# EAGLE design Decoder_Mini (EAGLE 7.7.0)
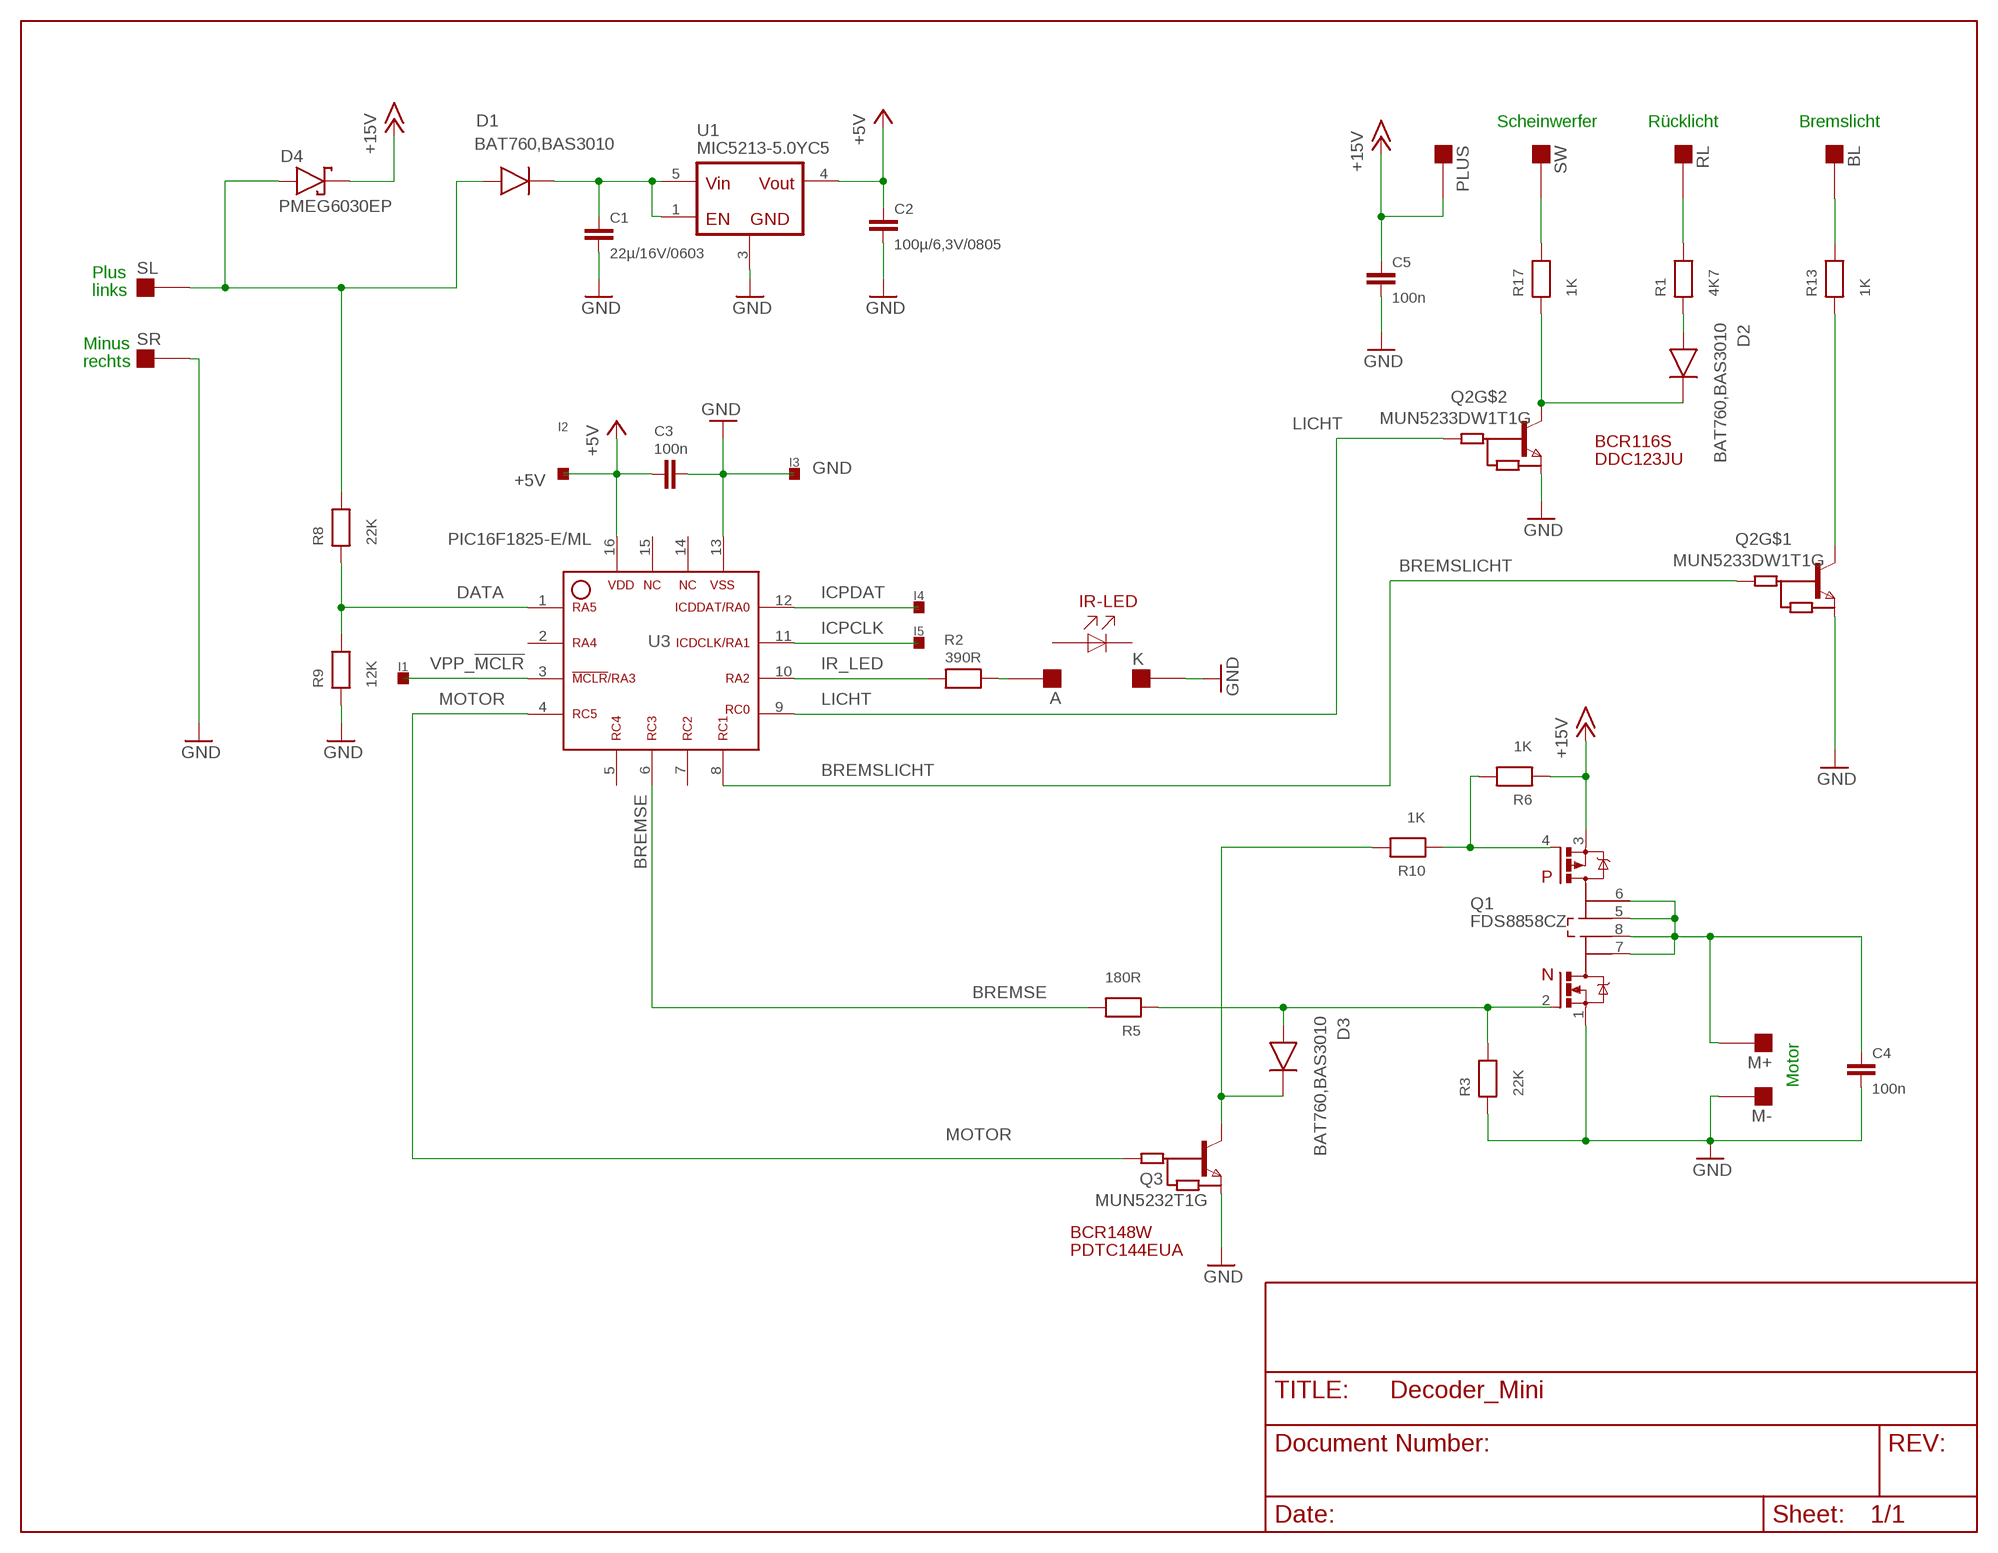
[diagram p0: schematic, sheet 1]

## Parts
A  A  LOETPAD1.5  [LOETPAD_RUND]
BL  LOETPAD_1.6X1.6_MM  [LOETPAD_1.6X1.6_MM]
C1  22µ/16V/0603  C-0603R  [0603-R]
C2  100µ/6,3V/0805  C-0805R  [0805-R]
C3  100n  C-0402R  [0402-R]
C4  100n  C-0402R  [0402-R]
C5  100n  C-0402R  [0402-R]
D1  BAT760,BAS3010  BAR65-03WBIG  [SOD323_BIG]
D2  BAT760,BAS3010  BAR65-03WBIG  [SOD323_BIG]
D3  BAT760,BAS3010  BAR65-03WBIG  [SOD323_BIG]
D4  PMEG6030EP  [SOD128]
I1  INCIR-PADOVAL  [TEST_PAD_OVAL]
I2  INCIR-PADOVAL  [TEST_PAD_OVAL]
I3  INCIR-PADOVAL  [TEST_PAD_OVAL]
I4  INCIR-PADOVAL  [TEST_PAD_OVAL]
I5  INCIR-PADOVAL  [TEST_PAD_OVAL]
K  K  LOETPAD1.5  [LOETPAD_RUND]
M+  LOETPAD_2X2MM  [LOETPAD_2X2_MM]
M-  LOETPAD_2X2MM  [LOETPAD_2X2_MM]
PLUS  LOETPAD_1.6X1.6_MM  [LOETPAD_1.6X1.6_MM]
Q1  FDS8858CZ  SI4501BDY  [SO8_COOLING]
Q2  MUN5233DW1T1G  DDC123JUSOT363-3  [SOT363-6]
Q3  MUN5232T1G  PDTC144EUFRANK  [SC70_FRANK]
R1  4K7  RES-0402W  [0402-W]
R2  390R  RES-0402R  [0402-R]
R3  22K  RES-0402R  [0402-R]
R5  180R  RES-0402W  [0402-W]
R6  1K  RES-0402W  [0402-W]
R8  22K  RES-0402R  [0402-R]
R9  12K  RES-0402R  [0402-R]
R10  1K  RES-0402W  [0402-W]
R13  1K  RES-0402W  [0402-W]
R17  1K  RES-0402W  [0402-W]
RL  LOETPAD_1.6X1.6_MM  [LOETPAD_1.6X1.6_MM]
SL  LOETPAD_2X2MM  [LOETPAD_2X2_MM]
SR  LOETPAD_2X2MM  [LOETPAD_2X2_MM]
SW  LOETPAD_1.6X1.6_MM  [LOETPAD_1.6X1.6_MM]
U1  MIC5213-5.0YC5  MIC5213  [SOT363-5]
U3  PIC16F1825-E/ML  PIC16F182X/ML  [QFN_4X4X0.9]

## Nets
+5V: C2.1 C3.1 I2.1 U1.4(VOUT) U3.16
+15V: C5.1 D4.K PLUS.P$1 Q1.3(S2) R6.1
AN: A.P$1 R2.1
BREMSE: R5.2 U3.6
BREMSLICHT: Q2.2(B) U3.8
D!: D2.K Q2.3(C) R17.1
DATA: R8.1 R9.2 U3.1
GND: C1.2 C2.2 C3.2 C4.2 C5.2 I3.1 K.P$1 M-.P$1 Q1.1(S1) Q2.1(E) Q2.4(E) Q3.2(E) R3.1 R9.1 SR.P$1 U1.3(GND) U3.13
ICPCLK: I5.1 U3.11
ICPDAT: I4.1 U3.12
IR_LED: R2.2 U3.10
LICHT: Q2.5(B) U3.9
M_PLUS: C4.1 M+.P$1 Q1.5(D2A) Q1.6(D2B) Q1.7(D1A) Q1.8(D1B)
MOTOR: Q3.1(B) U3.4
N$1: C1.1 D1.K U1.1(EN) U1.5(VIN)
N$4: BL.P$1 R13.2
N$6: D1.A D4.A R8.2 SL.P$1
N$7: R1.2 RL.P$1
N$8: D2.A R1.1
N$9: R17.2 SW.P$1
N$11: D3.A Q1.2(G1) R3.2 R5.1
N$13: Q2.6(C) R13.1
N$16: D3.K Q3.3(C) R10.2
N$17: Q1.4(G2) R6.2 R10.1
VPP_!MCLR!: I1.1 U3.3
Unconnected: U3.2 U3.5 U3.7 U3.14 U3.15

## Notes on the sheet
- Scheinwerfer | Rücklicht | Bremslicht
- Plus
- links
- Minus
- rechts
- BCR116S
- DDC123JU
- IR-LED
- Motor
- BCR148W
- PDTC144EUA

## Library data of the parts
A K = Hobby:LOETPAD: Lötpad
BL PLUS RL SW = Hobby:LOETPAD_1.6X1.6_MM: Lötpad 1,6 x 1,6 mm, Bohrung 0,7mm
C1-C5 = RCL:C: Kondensatoren CM 2003
D1-D3 = SMD:BAR65-03W*
D4 = Hobby:PMEG6030EP: 3 A low VF MEGA Schottky barrier rectifier
I1-I5 = SMD:INCIR-PAD*
M+ M- SL SR = Hobby:LOETPAD_2X2MM: Lötpad 2 x 2 mm mit Durchkontaktierung
Q1 = Hobby:SI4501BDY: Complementary N and P Channel MOSFET
Q2 = Hobby:DDC123JU*: NPN PRE-BIASED SMALL SIGNAL DUAL SURFACE MOUNT TRANSISTOR
Q3 = Hobby:PDTC144EU*: NPN Transistor mit Vorwiderständen
R1-R3 R5 R6 R8-R10 R13 R17 = RCL:RES: Widerstand
U1 = Hobby:MIC5213: Teeny™ SC-70 μCap Low-Dropout Regulator
U3 = Hobby:PIC16F182X*: Microchip 8 Bit µC

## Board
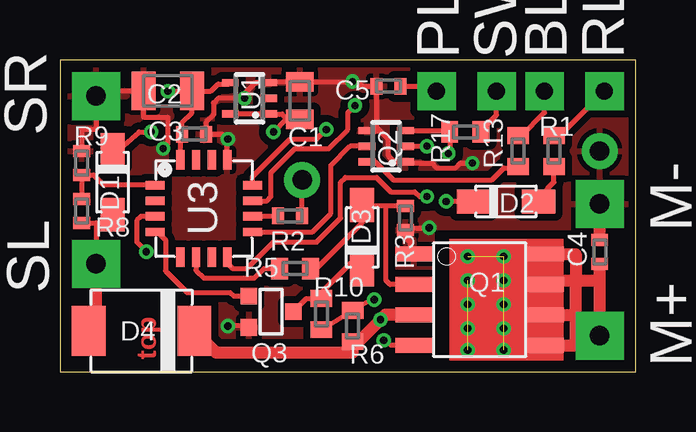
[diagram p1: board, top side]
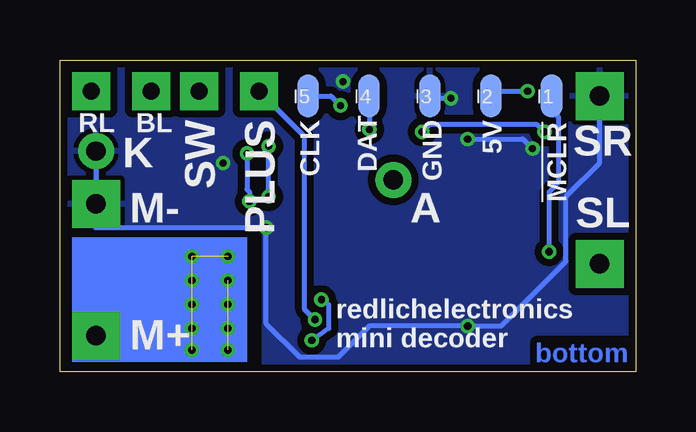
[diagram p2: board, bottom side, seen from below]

Size 24 x 13 mm. Coordinates in mm from the lower left corner, seen from the top.
Outline: 0,0 24,0 24,13 0,13 0,0
Copper layers (1*16): Top 0.035mm / dielectric 1.5mm / Bottom 0.035mm
Design rules "PCB-POOL Standard *": minimum track width 0.15mm, minimum drill 0.3mm, track to track 0.15mm, track to pad 0.15mm, pad to pad 0.15mm, via to via 0.15mm, smd to smd 0.15mm, copper to edge 0.3mm, drill to drill 0.2mm, minimum pad ring 0.2mm, minimum via ring 0.15mm, stop-mask expansion 0.075mm, vias tented up to drill 0.5mm, thermal gap 0.2mm

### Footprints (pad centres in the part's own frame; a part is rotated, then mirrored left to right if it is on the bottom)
LOETPAD_RUND = drill 0.8 pad 1.5: P$1 0,0
LOETPAD_1.6X1.6_MM = drill 0.7 pad 1.6 square: P$1 0,0
0603-R = smd 0.813 x 1.143: 1 -0.787,0; 2 0.787,0
0805-R = smd 0.991 x 1.6: 1 -1.016,0; 2 1.016,0
0402-R = smd 0.5 x 0.7: 1 -0.5,0; 2 0.5,0
SOD323_BIG = smd 1.4 x 1: A 1.35,0; K -1.35,0
SOD128 = smd 1.4 x 2.1: A -2.2,0; K 2.2,0
TEST_PAD_OVAL = smd 0.9 x 1.8: 1 0,0
LOETPAD_2X2_MM = drill 0.8 pad 2 square: P$1 0,0
SO8_COOLING = smd 0.61 x 1.524: 1 -1.905,-2.743; 2 -0.635,-2.743; 3 0.635,-2.743; 4 1.905,-2.743; 5 1.905,2.743; 6 0.635,2.743; 7 -0.635,2.743; 8 -1.905,2.743
SOT363-6 = smd 0.3 x 0.7: 1 -0.65,-0.8; 2 0,-0.8; 3 0.65,-0.8; 4 0.65,0.8; 5 0,0.8; 6 -0.65,0.8
SC70_FRANK = smd 0.7 x 0.7: 1 -0.65,-0.925; 2 0.65,-0.925; 3 0,0.925
0402-W = smd 0.7 x 0.9: 1 -0.65,0; 2 0.65,0
SOT363-5 = smd 0.3 x 0.7: 1 -0.65,-0.8; 2 0,-0.8; 3 0.65,-0.8; 4 0.65,0.8; 5 -0.65,0.8
QFN_4X4X0.9 = smd 0.35 x 0.8: 1 -0.975,-2.031; 2 -0.325,-2.031; 3 0.325,-2.031; 4 0.975,-2.031; 9 0.975,2.031; 10 0.325,2.031; 11 -0.325,2.031; 12 -0.975,2.031 | smd 0.8 x 0.35: 5 2.031,-0.975; 6 2.031,-0.325; 7 2.031,0.325; 8 2.031,0.975; 13 -2.031,0.975; 14 -2.031,0.325; 15 -2.031,-0.325; 16 -2.031,-0.975

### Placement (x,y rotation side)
A  10.1,8 0 top
BL  20.2,11.7 0 top
C1  10,11.3 90 top
C2  4.5,11.7 180 top
C3  5.6,9.9 0 top
C4  22.5,5 90 top
C5  13.7,11.9 180 top
D1  2.2,7.9 270 top
D2  18.6,7.1 0 top
D3  12.6,5.6 90 top
D4  3.4,1.7 0 top
I1  3.5,11.5 0 bottom
I2  6.04,11.5 0 bottom
I3  8.58,11.5 0 bottom
I4  11.12,11.5 0 bottom
I5  13.66,11.5 0 bottom
K  22.5,9.2 0 top
M+  22.5,1.5 270 top
M-  22.5,7 270 top
PLUS  15.7,11.7 0 top
Q1  17.5,3 270 top
Q2  13.6,9.4 90 top
Q3  8.8,2.5 270 top
R1  20.6,9.2 90 top
R2  9.6,6.5 180 top
R3  14.4,6.4 90 top
R5  9.8,4.3 180 top
R6  12.2,1.9 90 top
R8  0.9,6.7 270 top
R9  0.9,8.7 270 top
R10  10.9,2.4 90 top
R13  19.1,9.2 90 top
R17  16.9,10 0 top
RL  22.7,11.7 0 top
SL  1.5,4.5 0 top
SR  1.5,11.5 0 top
SW  18.2,11.7 0 top
U1  7.9,11.4 90 top
U3  6,6.8 270 top

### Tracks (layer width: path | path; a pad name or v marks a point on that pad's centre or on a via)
+5V  (via drill 0.3)
  Top 0.2: v4.5,11.7 C2.1 | C2.1 6.3,11.7 6.6,12 7.05,12 U1.4 | C2.1 5.5,11.68 5.5,10.8 5.1,10.4 C3.1 5.03,9.82 U3.16
  Bottom 0.2: I2.1 5.84,11.7 v4.5,11.7
+15V  (via drill 0.3)
  Top 0.2: C5.1 15.5,11.9 PLUS.P$1
  Top 0.5: D4.K 6.5,0.8 12.2,0.8 R6.1 12.45,1.25 v13.37,2.17 13.56,2.37 Q1.3
  Bottom 0.2: v13.37,2.17 13.8,2.6 13.8,9.8 PLUS.P$1
AN
  Top 0.2: R2.1 A.P$1
BREMSE
  Top 0.2: U3.6 5.67,4.22 6,3.9 8.1,3.9 8.5,4.3 R5.2
BREMSLICHT  (via drill 0.3)
  Top 0.2: U3.8 7.03,4.47 7.2,4.3 7.8,4.3 8.9,5.4 10.7,5.4 11.7,6.4 11.7,7.9 11.9,8.1 13.2,8.1 13.8,7.5 14.8,7.5 15,7.3 v15.3,7.3 | Q2.2 v15.3,9.4
  Bottom 0.2: v15.3,7.3 v15.3,9.4
D!  (via drill 0.3)
  Top 0.2: Q2.3 16.2,10.05 R17.1 16.25,9.25 v16.2,9.1 | D2.K v16.1,7.1
  Bottom 0.2: v16.2,9.1 16.2,7.6 16.1,7.5 v16.1,7.1
DATA
  Top 0.2: R8.1 R9.2 1.4,8.2 1.82,7.78 U3.1
GND  (via drill 0.3)
  Top 0.2: 0.91,9.21 R9.1 0.9,10.1 1.5,10.1 SR.P$1 1.7,11.7 C2.2 3.48,10.62 3.5,10.6 4.5,10.6 4.5,9.5 v4.3,9.3 | U3.13 6.97,9.68 v7,9.7 6.8,9.9 C3.2 6.1,10.4 6.4,10.7 6.4,11.2 6.6,11.4 v7.7,11.4 7.7,11.6 8.15,12.05 U1.3 8.74,12.09 C1.2 10.29,12.09 10.3,12.1 v12.2,12.1 12.4,12.1 12.6,11.9 C5.2 13.2,10.2 13.35,10.05 | Q3.2 7.65,1.85 7.6,1.9 v7,1.9 | Q1.1 14.6,5.06 14.6,5.4 14.4,5.6 R3.1 14.5,6 v15.4,6 | 12.9,10.05 Q2.4 13.35,10.05 | 13.35,10.05 13.7,9.7 13.7,9 13.95,8.75 Q2.1 14.45,8.7 15.5,8.7 15.7,8.5 16.5,8.5 16.7,8.7 v17.2,8.7
  Top 0.5: C4.2 M-.P$1
  Bottom 0.2: I3.1 8.48,11.4 v7.7,11.4 | v7,9.7 4.7,9.7 v4.3,9.3 | SR.P$1 1.5,8.7 2.9,7.3 2.9,4.6 5.6,1.9 v7,1.9 11.1,1.9 12.4,0.6 14,0.6 15.4,2 v15.4,6 22.5,6 M-.P$1 K.P$1
  pour Top (isolate 0.3): 0,13 24,13 24,6 15.5,6 15.5,0 0,0
  pour Bottom (isolate 0.3): 0,13 24,13 24,6 15.5,6 15.5,0 0,0
ICPCLK  (via drill 0.3)
  Top 0.2: U3.11 8.62,7.12 8.8,7.3 8.8,8.3 9.8,9.3 11.2,9.3 12,10.1 12,10.8 v12.3,11.1
  Bottom 0.2: I5.1 12.7,11.5 v12.3,11.1
ICPDAT  (via drill 0.3)
  Top 0.2: U3.12 8.03,8.13 9.6,9.7 10.7,9.7 v11.1,10.1
  Bottom 0.2: I4.1 11.12,10.72 11.1,10.7 v11.1,10.1
IR_LED
  Top 0.2: U3.10 8.06,6.5 R2.2
LICHT
  Top 0.2: U3.9 10.53,5.83 11.3,6.6 11.3,8.6 12.1,9.4 Q2.5
M_PLUS
  Top 0.2: Q1.7 20.41,3.8
  Top 0.5: M+.P$1 22.5,3.8 | 22.5,3.8 C4.1 | 20.41,3.8 21.5,3.8 | Q1.8 21.5,4.91 21.5,3.8 | Q1.6 21.5,2.37 | 21.5,2.37 21.5,3.8 | Q1.5 21.5,1.09 21.5,2.37 | 21.5,3.8 22.5,3.8
MOTOR
  Top 0.2: U3.4 4.08,5.83 4.4,5.5 4.4,4.2 5.3,3.3 7.1,3.3 7.25,3.15 Q3.1
N$1  (via drill 0.3)
  Top 0.2: D1.K 2.2,9.3 2.5,9.3 3.3,10 v3.8,10 | U1.5 U1.1 9.26,10.75 9.5,10.51 | C1.1 9.5,10.51 | 9.5,10.51 9.41,10.51 v8.9,10
  Bottom 0.2: v3.8,10 4.1,10.3 8.6,10.3 v8.9,10
N$2  (via drill 0.3)  (5 unrouted)
  other vias: 17,4.8 18.5,4.8 18.5,3.8 18.5,2.8 18.5,1.8 18.5,0.9
N$3  (via drill 0.3)  (3 unrouted)
  other vias: 17,3.8 17,2.8 17,1.8 17,0.9
N$4
  Top 0.2: R13.2 19.25,9.85 20.2,10.8 BL.P$1
N$6
  Top 0.2: R8.2 1.5,6.2 | 1.5,6.2 SL.P$1 | 1.5,6.2 2.4,6.2 D1.A
  Top 0.5: D4.A 1.5,2 SL.P$1
N$7
  Top 0.2: R1.2 20.85,9.85 RL.P$1
N$8
  Top 0.2: D2.A 20.35,7.65 20.6,7.9 R1.1
N$9
  Top 0.2: R17.2 17.55,10.05 18.2,10.7 SW.P$1
N$11
  Top 0.2: R5.1 10.7,4.3 12.6,6.2 D3.A 12.95,6.9 13.6,6.9 | Q1.2 13.77,3.63 13.6,3.8 13.6,6.9 | R3.2 13.6,6.9
N$13
  Top 0.2: Q2.6 13.15,8.75 13.9,8 18,8 18.5,8.5 19.05,8.5 R13.1
N$16
  Top 0.2: Q3.3 10.28,3.05 R10.2 10.9,3.3 12.15,4.55 D3.K
N$17  (via drill 0.3)
  Top 0.2: R10.1 R6.2 13.05,3.05 v13.1,3 | Q1.4 13.79,1.09 v13.5,1.3
  Bottom 0.2: v13.1,3 12.8,2.8 12.8,1.8 v13.5,1.3
VPP_!MCLR!  (via drill 0.3)
  Top 0.2: U3.3 3.38,6.47 3.2,6.3 3.2,5.5 3.2,5.4 v3.6,5
  Bottom 0.2: v3.6,5 3.6,7.5 3.2,7.9 3.2,10.6 3.4,10.8 3.4,11.4 I1.1
(copper drawn outside any net)
  shapes: Bottom area x1

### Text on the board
Top: top
Bottom: bottom
Document: Decoder DIY Rev.2.1 / / SL Slot Links / SR Slot Rechts / A IR-LED Anode / K IR-LED Kathode / BL LED (2 in Reihe) Bremslicht Kathode / RL LED (2 in Reihe) Rücklicht Kathode / SW LED (2 in Reihe) Scheinwerfer Kathode / PLUS LED Rück-,Bremslicht und Scheinwerfer Anode / / PROG_1 PICkit3 Pin1 !MCLR! / PROG_2 PICkit3 Pin2 5V / PROG_3 PICkit3 Pin3 GND / PROG_4 PICkit3 Pin4 DAT / PROG_5 PICkit3 Pin5 CLK / n.c. PICkit3 Pin6 frei
bSilk: DAT | BL | RL | !MCLR! | 5V | GND | CLK | PLUS | SW | SR | K | SL | A | M- | redlichelectronics / mini decoder | M+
